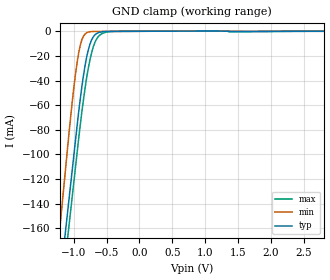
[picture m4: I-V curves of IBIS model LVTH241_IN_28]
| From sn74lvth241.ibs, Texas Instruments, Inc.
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[Model]   LVTH241_IN_28
Model_type  Input
Vinl = 0.8
Vinh = 2.0
| variable   typ   min   max
C_comp   3.89pF   3.15pF   5.27pF
[Temperature Range]   40   -40   100
| Ambient temperature   25   -40   85
[Voltage range]   2.8   2.7   2.9
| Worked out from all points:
|   GND clamp passes 1 mA (typ) near -0.62 V on its own axis
[GND Clamp]
| LVTH241_IN_28
|   Voltage   I(typ)   I(min)   I(max)
-5.5V     -2.408A    -2.65A     -2.407A
-1.22V    -209.4mA   -166.2mA   -230.2mA
-1.205V   -202.1mA   -157.8mA   -222.9mA
-1.125V   -163.2mA   -113.2mA   -184.4mA
-1.075V   -138.9mA   -85.42mA   -160.3mA
-975mV    -90.32mA   -36.3mA    -112.1mA
-900mV    -55.42mA   -11.62mA   -76.6mA
-800mV    -20.4mA    -1.145mA   -37.03mA
-675mV    -2.832mA   -140.1uA   -8.833mA
-575mV    -458.4uA   -111.8uA   -2.088mA
-425mV    -91.65uA   -80.29uA   -190.6uA
2.8V      16.5pA     10.34pA    -1.624nA
